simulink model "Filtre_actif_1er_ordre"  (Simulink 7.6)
settings: Solver=ode15s  StartTime=0.0  StopTime=5  RelTol=1e-3
libraries: fl_lib x12, nesl_utility x4, simulink x1, elec_lib x1

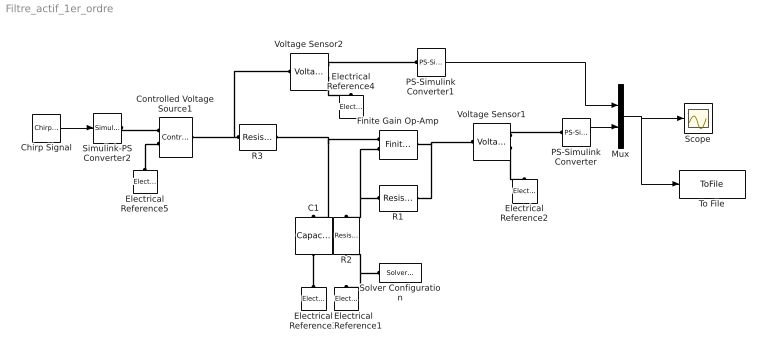
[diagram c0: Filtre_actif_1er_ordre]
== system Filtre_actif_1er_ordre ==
  C1 : fl_lib/Electrical/Electrical Elements/Capacitor  DialogController=NetworkEngine.DynNeDlgSource  SystemSampleTime=-1  c=1e-9 F  v0=0 V  r=1e-12 Ohm  g=0 1/Ohm  i_Log=off  v_Log=off  vc_Log=off  LocalVarNames=|current|voltage|power  LocalVarDescs=|Capacitor current (A)|Voltage across capacitor (V)|Power (W)  LocalVarLogging=[0 0 0]
  Chirp Signal : simulink/Sources/Chirp Signal  SystemSampleTime=-1  f1=10  T=1  f2=1000
  Controlled Voltage Source1 : fl_lib/Electrical/Electrical Sources/Controlled Voltage Source  DialogController=NetworkEngine.DynNeDlgSource  SystemSampleTime=-1  i_Log=off  v_Log=off  LocalVarNames=|current|voltage|power  LocalVarDescs=|Current (A)|Voltage (V)|Power (W)  LocalVarLogging=[0 0 0]
  Electrical Reference{1..5} (5 alike) : fl_lib/Electrical/Electrical Elements/Electrical Reference  DialogController=NetworkEngine.DynNeDlgSource  SystemSampleTime=-1  i_Log=off  LocalVarNames=|i  LocalVarDescs=|i  LocalVarLogging=[]
  Finite Gain Op-Amp : elec_lib/Integrated Circuits/Finite Gain Op-Amp  DialogController=NetworkEngine.DynNeDlgSource  SystemSampleTime=-1  A=1000  Rin=1e+06 Ohm  Rout=100 Ohm  Vmin=-15 V  Vmax=15 V  LocalVarNames=|power  LocalVarDescs=|Dissipated power (W)  LocalVarLogging=0
  Mux : Mux  Inputs=2
  PS-Simulink Converter : nesl_utility/PS-Simulink Converter  DialogController=NetworkEngine.DynNeUtilDlgSource  SystemSampleTime=-1  PhysicalDomain=network_engine_domain  LeftPortType=input  RightPortType=output  SubClassName=ps_output  Unit=1  AffineConversion=off
  PS-Simulink Converter1 : nesl_utility/PS-Simulink Converter  DialogController=NetworkEngine.DynNeUtilDlgSource  SystemSampleTime=-1  PhysicalDomain=network_engine_domain  LeftPortType=input  RightPortType=output  SubClassName=ps_output  Unit=1  AffineConversion=off
  R1 : fl_lib/Electrical/Electrical Elements/Resistor  DialogController=NetworkEngine.DynNeDlgSource  SystemSampleTime=-1  R=10e3 Ohm  i_Log=off  v_Log=off  LocalVarNames=|current|voltage|power  LocalVarDescs=|Resistor current (A)|Voltage across resistor (V)|Power (W)  LocalVarLogging=[0 0 0]
  R2 : fl_lib/Electrical/Electrical Elements/Resistor  DialogController=NetworkEngine.DynNeDlgSource  SystemSampleTime=-1  R=10e3 Ohm  i_Log=off  v_Log=off  LocalVarNames=|current|voltage|power  LocalVarDescs=|Resistor current (A)|Voltage across resistor (V)|Power (W)  LocalVarLogging=[0 0 0]
  R3 : fl_lib/Electrical/Electrical Elements/Resistor  DialogController=NetworkEngine.DynNeDlgSource  SystemSampleTime=-1  R=100e3 Ohm  i_Log=off  v_Log=off  LocalVarNames=|current|voltage|power  LocalVarDescs=|Resistor current (A)|Voltage across resistor (V)|Power (W)  LocalVarLogging=[0 0 0]
  Scope : Scope
  Simulink-PS Converter2 : nesl_utility/Simulink-PS Converter  DialogController=NetworkEngine.DynNeUtilDlgSource  SystemSampleTime=-1  PhysicalDomain=network_engine_domain  LeftPortType=input  RightPortType=output  SubClassName=ps_input  Unit=1  AffineConversion=off  InputFilterTimeConstant=.001  UdotUserProvided=0
  Solver Configuration : nesl_utility/Solver Configuration  DialogController=NetworkEngine.DynNeUtilDlgSource  SystemSampleTime=-1  PhysicalDomain=network_engine_domain  LeftPortType=input  RightPortType=generic  SubClassName=solver  Accelerate=off  Profile=off  ResidualTolerance=1e-40  MaxNonlinIter=12  MaxModeIter=2  DoFixedCost=off  UseLocalSampling=off  DoDC=on  LinearAlgebra=Full  LocalSolverSampleTime=.001  LocalSolverChoice=NE_BACKWARD_EULER_ADVANCER  UseLocalSolver=off
  To File : ToFile  Filename=filtre_1ordre  MatrixName=xy
  Voltage Sensor1 : fl_lib/Electrical/Electrical Sensors/Voltage Sensor  DialogController=NetworkEngine.DynNeDlgSource  SystemSampleTime=-1  i1_Log=off  v1_Log=off  LocalVarNames=|i1|v1  LocalVarDescs=|i1|v1  LocalVarLogging=[]
  Voltage Sensor2 : fl_lib/Electrical/Electrical Sensors/Voltage Sensor  DialogController=NetworkEngine.DynNeDlgSource  SystemSampleTime=-1  i1_Log=off  v1_Log=off  LocalVarNames=|i1|v1  LocalVarDescs=|i1|v1  LocalVarLogging=[]
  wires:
  PS-Simulink Converter/1 -> Mux/2
  Mux/1 -> Scope/1, To File/1
  PS-Simulink Converter1/1 -> Mux/1
  Chirp Signal/1 -> Simulink-PS Converter2/1
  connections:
  Voltage Sensor1/RConn1 -- PS-Simulink Converter/LConn1
  Voltage Sensor1/RConn2 -- Electrical Reference2/LConn1
  R1/LConn1 -- Finite Gain Op-Amp/RConn1 -- Voltage Sensor1/LConn1
  R1/RConn1 -- Finite Gain Op-Amp/LConn2 -- R2/LConn1
  C1/LConn1 -- Electrical Reference3/LConn1
  Finite Gain Op-Amp/LConn1 -- C1/RConn1 -- R3/LConn1
  Solver Configuration/RConn1 -- R2/RConn1 -- Electrical Reference1/LConn1
  Voltage Sensor2/LConn1 -- R3/RConn1 -- Controlled Voltage Source1/LConn1
  Voltage Sensor2/RConn1 -- PS-Simulink Converter1/LConn1
  Voltage Sensor2/RConn2 -- Electrical Reference4/LConn1
  Simulink-PS Converter2/RConn1 -- Controlled Voltage Source1/RConn1
  Electrical Reference5/LConn1 -- Controlled Voltage Source1/RConn2
